|//////////////////////////////////////////////////////////////////////////////
|//////////////////////////////////////////////////////////////////////////////
|   @@@@@@@   @@@@@@@   @@@@@@@   @@@@@@@   @@@@@@@   @@@@@@   @@
|   @@@@@@@@@   @@@@@@@@@   @@@@@@@@@   @@@@@@@@@   @@@@@@@@@ @@@@@@@@  @
|   @@@   @@@ @@@   @@@ @@@   @@@   @@@ @@@   @@@@   @@@  @
|   @@   @@ @@   @@ @@@@@@@@@@@ @@@@@@@@@@@ @@   @@   @@ @@
|   @@@   @@@ @@   @@   @@@ @@@   @@   @@   @@ @@
|   @@@@@@@@@  @@   @@  @@@@@@@@@   @@@@@@@@@  @@   @@   @@ @@
|   @@@@@@@   @@   @@   @@@@@@@   @@@@@@@   @@   @@   @@ @@
|   IBIS Model of NL17SZ125
|   Non-Inverting 3-State Buffer
|   Package Type: SC-74A (DBV), CASE 318BQ
|   SC-88A / SC-70-5 (DF), CASE 419A-02
|   SOT-953, CASE 527AE (P5)
|   SOT-553 (XV5), CASE 463B-01
|   UDFN6, CASE 517AQ (1.45 x 1.00 mm)
|   UDFN6, CASE 517BX (1.00 x 1.00 mm)
|   The model is covering the following Vccs:
|   1.8V, 2.5V, 3.3V, 5.0V
|//////////////////////////////////////////////////////////////////////////////
|//////////////////////////////////////////////////////////////////////////////
[IBIS Ver]   3.2
|   7.2 compatible
|//////////////////////////////////////////////////////////////////////////////
[Comment Char] |_char
|//////////////////////////////////////////////////////////////////////////////
[File Name]   nl17sz125_va_r0.ibs
|//////////////////////////////////////////////////////////////////////////////
[File Rev]   0.0
|   0.0 - Jan 15, 2025 - File created
|//////////////////////////////////////////////////////////////////////////////
[Date]   January 15, 2025
|//////////////////////////////////////////////////////////////////////////////
[Source]   From lab measurements and simulations at onsemi
|//////////////////////////////////////////////////////////////////////////////
[Notes]
   - The currents greater than +/- 100 mA are extrapolated
|//////////////////////////////////////////////////////////////////////////////
[Disclaimer]
   - onsemi Corporation hereby grants
   the user of this IBIS model a license to use this model
   under the following terms. This license is nonexclusive
   and nontransferable. Before using this IBIS model.
   After reading the terms and conditions of this license,
   the user either must accept these terms,
   or the IBIS model should be returned to onsemi within 30 days.
   - The user is hereby granted a license to use the IBIS model.
   This shall not be construed as a right to sell,
   or otherwise profit either by leasing or renting this software.
   - The user may modify the IBIS model to suit his specific
   applications but rights to derivative works and such
   modifications shall belong to onsemi.
   - This IBIS model is provided on an "as is" basis.
   onsemi makes absolutely no warranty with respect
   to the information contained herein.
   By use of this IBIS model, the user assumes full risk as to the
   quality and suitablility of the model to his particular use,
   and by using this model assumes the entire risk.
   Under all circumstances the user shall not hold
   onsemi liable in any way for the results obtained.
   onsemi reserves the right to make to improve
   the model for reliability, function, or design.
   onsemi does not convey any license under patent
   rights or any other intellectual property rights,
   including those of third parties.
   - onsemi is not obligated to provide maintenance
   or support for the licensed IBIS model.
   - Cont onsemi at ATTN:LOGIC APPLICATIONS/IBIS MODEL.
   5701 N Pima Rd, Scottsdale, AZ 85250
|//////////////////////////////////////////////////////////////////////////////
[Copyright]   (c) 2025 onsemi Corp.
|//////////////////////////////////////////////////////////////////////////////
|//////////////////////////////////////////////////////////////////////////////
[Component]   NL17SZ125P5T5G
|//////////////////////////////////////////////////////////////////////////////
[Manufacturer]  onsemi
|   Data Sheet: NL17SZ125/D, Rev. 25,  May, 2023
|//////////////////////////////////////////////////////////////////////////////
[Package]
|  SOT-953
| P5  SUFFIX
| CASE 527AE
| variable   typ   min   max
R_pkg   0.0786   0.0731   0.0817
L_pkg   1.1377nH   1.0330nH   1.1757nH
C_pkg   0.0487pF   0.0295pF   0.0642pF
|//////////////////////////////////////////////////////////////////////////////
[Pin]   signal_name   model_name   R_pin   L_pin   C_pin
1   A   In   0.0817   1.1757nH   0.0433pF
2   GND   GND   0.0731   1.0330nH   0.0295pF
3   OE   In   0.0805   1.1531nH   0.0500pF
4   Y   Out   0.0789   1.1637nH   0.0642pF
5   VCC   POWER   0.0787   1.1630nH   0.0567pF
|//////////////////////////////////////////////////////////////////////////////
|//////////////////////////////////////////////////////////////////////////////
[Component]   NL17SZ125DBVT1G
|//////////////////////////////////////////////////////////////////////////////
[Manufacturer]  onsemi
|   Data Sheet: NL17SZ125/D, Rev. 25,  May, 2023
|//////////////////////////////////////////////////////////////////////////////
[Package]
|  SC-74A
| DBV SUFFIX
| CASE 318BQ
| variable   typ   min   max
R_pkg   0.0710   0.0522   0.0935
L_pkg   1.2331nH   1.0634nH   1.4484nH
C_pkg   0.1280pF   0.1167pF   0.1367pF
|//////////////////////////////////////////////////////////////////////////////
[Pin]   signal_name   model_name   R_pin   L_pin   C_pin
1   OE   In   0.0522   1.0634nH   0.1235pF
2   A   In   0.0588   1.1995nH   0.1367pF
3   GND   GND   0.0828   1.3327nH   0.1351pF
4   Y   Out   0.0935   1.4484nH   0.1279pF
5   VCC   POWER   0.0679   1.1215nH   0.1167pF
|//////////////////////////////////////////////////////////////////////////////
|//////////////////////////////////////////////////////////////////////////////
|[Component]   NL17SZ125DTT1G
||//////////////////////////////////////////////////////////////////////////////
|[Manufacturer]  onsemi
||   Data Sheet: NL17SZ125/D, Rev. 25,  May, 2023
||//////////////////////////////////////////////////////////////////////////////
|[Package]
|| TSOP-5/SOT-23-5
||   DT SUFFIX
||   CASE 483
|| variable   typ   min   max
|R_pkg   0.02532   0.0216   0.0295
|L_pkg   1.52928nH   1.3125nH   1.9067nH
|C_pkg   0.15688pF   0.1108pF   0.2403pF
||//////////////////////////////////////////////////////////////////////////////
|[Pin]   signal_name   model_name   R_pin   L_pin   C_pin
|1   OE   In   0.0216   1.5112nH   0.1443pF
|2   A   In   0.0237   1.3125nH   0.1382pF
|3   GND   GND   0.0295   1.9067nH   0.2403pF
|4   Y   Out   0.0266   1.5415nH   0.1508pF
|5   VCC   POWER   0.0252   1.3745nH   0.1108pF
|//////////////////////////////////////////////////////////////////////////////
|//////////////////////////////////////////////////////////////////////////////
[Component]   NL17SZ125XV5T2G
|//////////////////////////////////////////////////////////////////////////////
[Manufacturer]  onsemi
|   Data Sheet: NL17SZ125/D, Rev. 25,  May, 2023
|//////////////////////////////////////////////////////////////////////////////
[Package]
|  SOT-553
| XV5 SUFFIX
| CASE 463B-01
| variable   typ   min   max
R_pkg   0.0321   0.0287   0.0357
L_pkg   0.9169nH   0.7230nH   1.1357nH
C_pkg   0.2220pF   0.1035pF   0.3741pF
|//////////////////////////////////////////////////////////////////////////////
[Pin]   signal_name   model_name   R_pin   L_pin   C_pin
1   OE   In   0.0341   0.7230nH   0.1035pF
2   A   In   0.0287   0.8933nH   0.2377pF
3   GND   GND   0.0290   1.0725nH   0.3741pF
4   Y   Out   0.0357   0.7602nH   0.1139pF
5   VCC   POWER   0.0330   1.1357nH   0.2807pF
|//////////////////////////////////////////////////////////////////////////////
|//////////////////////////////////////////////////////////////////////////////
[Component]   NL17SZ125DFT2G
|//////////////////////////////////////////////////////////////////////////////
[Manufacturer]  onsemi
|   Data Sheet: NL17SZ125/D, Rev. 25,  May, 2023
|//////////////////////////////////////////////////////////////////////////////
[Package]
| SC-88A / SC-70-5
|   DF SUFFIX
|   CASE 419A-02
| variable   typ   min   max
R_pkg   0.0201   0.0170   0.0250
L_pkg   0.9982nH   0.8810nH   1.0690nH
C_pkg   0.1466pF   0.1187pF   0.2051pF
|//////////////////////////////////////////////////////////////////////////////
[Pin]   signal_name   model_name   R_pin   L_pin   C_pin
1   OE   In   0.0191   1.0690nH   0.1625pF
2   A   In   0.0187   0.8810nH   0.1217pF
3   GND   GND   0.0170   1.0315nH   0.2051pF
4   Y   Out   0.0207   0.9600nH   0.1249pF
5   VCC   POWER   0.0250   1.0497nH   0.1187pF
|//////////////////////////////////////////////////////////////////////////////
|//////////////////////////////////////////////////////////////////////////////
[Component]   NL17SZ125DFT2G-Q
|//////////////////////////////////////////////////////////////////////////////
[Manufacturer]  onsemi
|   Data Sheet: NL17SZ125/D, Rev. 25,  May, 2023
|//////////////////////////////////////////////////////////////////////////////
[Package]
R_pkg   0.0201   0.0170   0.0250
L_pkg   0.9982nH   0.8810nH   1.0690nH
C_pkg   0.1466pF   0.1187pF   0.2051pF
|//////////////////////////////////////////////////////////////////////////////
[Pin]   signal_name   model_name   R_pin   L_pin   C_pin
1   OE   In   0.0191   1.0690nH   0.1625pF
2   A   In   0.0187   0.8810nH   0.1217pF
3   GND   GND   0.0170   1.0315nH   0.2051pF
4   Y   Out   0.0207   0.9600nH   0.1249pF
5   VCC   POWER   0.0250   1.0497nH   0.1187pF
|//////////////////////////////////////////////////////////////////////////////
|//////////////////////////////////////////////////////////////////////////////
[Component]   NL17SZ125DFT1G-Q
|//////////////////////////////////////////////////////////////////////////////
[Manufacturer]  onsemi
|   Data Sheet: NL17SZ125/D, Rev. 25,  May, 2023
|//////////////////////////////////////////////////////////////////////////////
[Package]
R_pkg   0.0201   0.0170   0.0250
L_pkg   0.9982nH   0.8810nH   1.0690nH
C_pkg   0.1466pF   0.1187pF   0.2051pF
|//////////////////////////////////////////////////////////////////////////////
[Pin]   signal_name   model_name   R_pin   L_pin   C_pin
1   OE   In   0.0191   1.0690nH   0.1625pF
2   A   In   0.0187   0.8810nH   0.1217pF
3   GND   GND   0.0170   1.0315nH   0.2051pF
4   Y   Out   0.0207   0.9600nH   0.1249pF
5   VCC   POWER   0.0250   1.0497nH   0.1187pF
|//////////////////////////////////////////////////////////////////////////////
|//////////////////////////////////////////////////////////////////////////////
[Component]   NL17SZ125MU1TCG
|//////////////////////////////////////////////////////////////////////////////
[Manufacturer]  onsemi
|   Data Sheet: NL17SZ125/D, Rev. 25,  May, 2023
|//////////////////////////////////////////////////////////////////////////////
[Package]
|   UDFN-6
| 1.45 x 1.0
| CASE 517AQ
| variable   typ   min   max
R_pkg   0.0499   0.0010   0.0568
L_pkg   0.4063nH   0.0145nH   0.4786nH
C_pkg   0.1074pF   0.0765pF   0.1119pF
|//////////////////////////////////////////////////////////////////////////////
[Pin]   signal_name   model_name   R_pin   L_pin   C_pin
1   OE   In   0.0568   0.4786nH   0.1119pF
2   A   In   0.0469   0.3812nH   0.1077pF
3   GND   GND   0.0541   0.4521nH   0.1099pF
4   Y   Out   0.0513   0.4206nH   0.1072pF
5   NC   NC   0.0010   0.0145nH   0.0765pF
6   VCC   POWER   0.0484   0.3921nH   0.1051pF
|//////////////////////////////////////////////////////////////////////////////
|//////////////////////////////////////////////////////////////////////////////
[Component]   NL17SZ125MU3TCG
|//////////////////////////////////////////////////////////////////////////////
[Manufacturer]  onsemi
|   Data Sheet: NL17SZ125/D, Rev. 25,  May, 2023
|//////////////////////////////////////////////////////////////////////////////
[Package]
|  UDFN-6
| 1.0 x 1.0
| CASE 517BX
| variable   typ   min   max
R_pkg   0.0419   0.0344   0.0490
L_pkg   0.4237nH   0.3470nH   0.5107nH
C_pkg   0.1104pF   0.1061pF   0.1153pF
|//////////////////////////////////////////////////////////////////////////////
[Pin]   signal_name   model_name   R_pin   L_pin   C_pin
1   OE   In   0.0421   0.4133nH   0.1099pF
2   A   In   0.0344   0.3470nH   0.1061pF
3   GND   GND   0.0443   0.4580nH   0.1121pF
4   Y   Out   0.0490   0.5107nH   0.1153pF
5   NC   NC   0.0004   0.0379nH   0.0765pF
6   VCC   POWER   0.0438   0.4489nH   0.1118pF
|//////////////////////////////////////////////////////////////////////////////
|//////////////////////////////////////////////////////////////////////////////
[Model Selector]   In
In_18   Vcc = 1.80
In_25   Vcc = 2.50
In_33   Vcc = 3.30
In_50   Vcc = 5.00
|//////////////////////////////////////////////////////////////////////////////
[Model Selector]   Out
Out_18   Vcc = 1.80
Out_25   Vcc = 2.50
Out_33   Vcc = 3.30
Out_50   Vcc = 5.00
| Models and submodels in the file (8): In_18 (Input), Out_18 (3-state), In_25 (Input), Out_25 (3-state), In_33 (Input), Out_33 (3-state), In_50 (Input), Out_50 (3-state)
